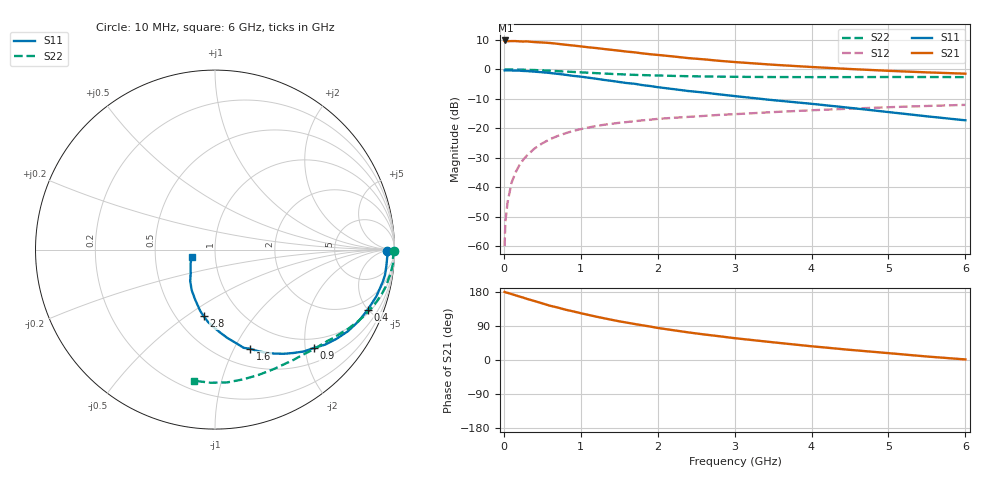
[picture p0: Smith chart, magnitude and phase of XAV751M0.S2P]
! SIEMENS Discrete & RF Semiconductors
! BFY180
! Si NPN RF Bipolar Junction Transistor in MICRO-X
! VCE = 0.75 V  IC = 1 mA
! Common Emitter S-Parameters:  May  1997
# GHz  S  MA  R  50
!  f  S11  S21  S12  S22
! GHz  MAG  ANG  MAG  ANG  MAG  ANG  MAG  ANG
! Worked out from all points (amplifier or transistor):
!   36 points, 10 MHz to 6 GHz, reference 50 ohm
!   highest |S21| = 9.8 dB at 20 MHz (marker M1)
!   |S21| within 3 dB of that: start of sweep to 1.336 GHz
!   unconditionally stable (mu >= 1): 2.765 GHz to end of sweep
!   at 250 MHz: K = 0.09, MSG = 20.1 dB, |S12| = -30.7 dB
!   at 1.4 GHz: K = 0.64, MSG = 12.6 dB, |S12| = -18.5 dB
!   at 6 GHz: K = 1.16, MAG = 2.9 dB, |S12| = -12.0 dB
!   S11 on the Smith chart (normalised r, x): 10 MHz: 48, -8; 400 MHz: 1.22, -5.00; 900 MHz: 0.79, -2.19; 1.6 GHz: 0.69, -1.16; 2.8 GHz: 0.68, -0.59; 6 GHz: 0.77, -0.06
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0.01  0.9605 -0.4  3.007 179.7  0.001 90.8  0.9956 -0.3
0.02  0.9663 -1.0  3.098 178.6  0.0026 90.3  0.9999 -0.7
0.05  0.9604 -2.5  3.012 177.2  0.0057 87.1  0.9952 -1.5
0.1  0.9592 -5.3  3.021 174.0  0.0119 88.9  0.9923 -3.0
0.15  0.9576 -8.5  3.025 170.9  0.0176 84.8  0.9945 -4.6
0.25  0.9422 -13.8  2.972 164.7  0.0291 81.9  0.9885 -7.6
0.3  0.9361 -16.2  2.984 161.3  0.0346 78.9  0.9823 -9.1
0.4  0.9148 -21.4  2.905 155.5  0.0456 75.0  0.9749 -11.9
0.6  0.8693 -31.5  2.805 143.2  0.0654 68.4  0.949 -17.3
0.8  0.8104 -40.8  2.623 132.8  0.0822 62.0  0.919 -22.2
0.9  0.7772 -44.8  2.543 128.4  0.0902 58.8  0.9054 -24.5
1.1  0.7231 -52.8  2.371 119.0  0.1032 54.1  0.8773 -28.5
1.3  0.6632 -60.8  2.22 110.3  0.1148 49.7  0.8508 -32.4
1.6  0.586 -70.5  2.002 98.6  0.1279 44.9  0.8182 -37.5
2  0.4989 -81.8  1.761 84.6  0.1446 39.3  0.7883 -43.6
2.2  0.4636 -86.4  1.659 78.7  0.1507 36.8  0.7757 -46.6
2.6  0.405 -95.5  1.482 67.5  0.1622 33.1  0.7588 -52.0
2.8  0.377 -99.6  1.399 62.7  0.169 31.3  0.754 -54.7
3.5  0.3006 -111.5  1.2 46.7  0.1885 25.6  0.7418 -63.9
4.5  0.2227 -128.4  1.015 26.8  0.2156 17.3  0.7398 -77.6
5.5  0.1599 -148.5  0.89 9.2  0.2395 9.0  0.7423 -91.9
6  0.1367 -163.2  0.846 1.5  0.2501 4.4  0.7397 -99.1
